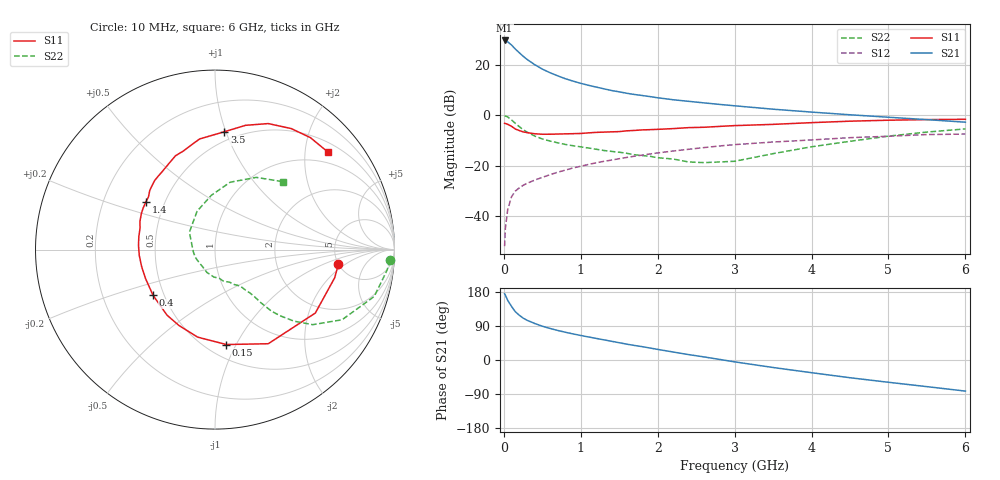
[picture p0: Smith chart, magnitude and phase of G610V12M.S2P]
! SIEMENS Small Signal Semiconductors
! BFG193
! Si NPN RF Bipolar Junction Transistor in SOT223
! VCE = 10 V  IC = 12 mA
! Common Emitter S-Parameters:  August  1996
# GHz  S  MA  R  50
!  f  S11  S21  S12  S22
! GHz  MAG  ANG  MAG  ANG  MAG  ANG  MAG  ANG
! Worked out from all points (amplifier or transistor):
!   36 points, 10 MHz to 6 GHz, reference 50 ohm
!   highest |S21| = 29.7 dB at 10 MHz (marker M1)
!   |S21| within 3 dB of that: start of sweep to 136.8 MHz
!   unconditionally stable (mu >= 1): 893 MHz to 2.527 GHz
!   at 250 MHz: K = 0.58, MSG = 25.7 dB, |S12| = -27.9 dB
!   at 1.4 GHz: K = 1.06, MAG = 12.3 dB, |S12| = -17.8 dB
!   at 6 GHz: K = 0.86, MSG = 2.4 dB, |S12| = -7.5 dB
!   S11 on the Smith chart (normalised r, x): 10 MHz: 5.01, -1.53; 150 MHz: 0.62, -0.91; 400 MHz: 0.44, -0.27; 1.4 GHz: 0.39, +0.27; 3.5 GHz: 0.43, +0.99; 6 GHz: 0.71, +2.51
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0.01  0.6923 -6.6  30.66 174.9  0.0025 84.5  0.9768 -3.4
0.02  0.6852 -13.2  30.3 171.1  0.0057 85.5  0.9658 -6.8
0.05  0.6613 -32.3  28.76 157.6  0.0133 75.2  0.9247 -16.4
0.1  0.6026 -60.5  24.88 141.4  0.024 66.0  0.8087 -28.9
0.15  0.5326 -83.2  20.67 127.3  0.0312 58.8  0.687 -37.5
0.2  0.4972 -101.2  17.55 118.3  0.0359 55.6  0.5952 -42.1
0.25  0.4683 -115.3  14.94 110.7  0.0404 52.9  0.5165 -45.5
0.3  0.4527 -126.2  12.94 105.0  0.0443 52.9  0.4642 -47.5
0.4  0.4289 -143.7  10.15 96.5  0.0513 53.0  0.3865 -49.3
0.5  0.4192 -157.4  8.268 89.1  0.0583 52.9  0.3381 -50.1
0.6  0.4197 -167.2  7.008 83.3  0.0659 53.7  0.3074 -51.3
0.7  0.4232 -175.6  6.073 78.0  0.0738 54.1  0.2834 -52.9
0.9  0.4305 170.3  4.768 68.8  0.0898 53.1  0.2478 -55.2
1.1  0.4466 159.5  3.937 60.8  0.1052 51.7  0.2233 -61.0
1.4  0.4681 145.1  3.104 49.4  0.1285 48.0  0.1911 -69.7
1.7  0.4994 134.8  2.585 38.3  0.1535 43.8  0.164 -80.5
2.2  0.5428 118.5  2.034 21.1  0.1945 34.6  0.135 -109.4
2.8  0.6001 102.2  1.645 1.7  0.2448 22.5  0.1178 -158.4
3.5  0.6589 85.4  1.319 -19.8  0.2937 6.6  0.1726 145.7
4.5  0.7622 67.1  1.022 -46.8  0.3585 -13.0  0.3035 93.8
5.5  0.8195 49.6  0.818 -70.3  0.4134 -37.0  0.4632 60.3
6  0.8315 40.8  0.728 -82.1  0.4223 -50.9  0.5353 45.0
